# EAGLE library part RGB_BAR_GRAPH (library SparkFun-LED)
SparkFun 48 Segment RGB Bar Graph - Common Anode
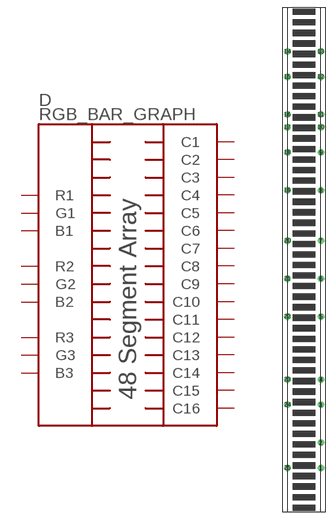
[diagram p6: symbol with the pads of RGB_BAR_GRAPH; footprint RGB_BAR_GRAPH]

Designator prefix D

## RGB_BAR_GRAPHCA (PROD_ID: COM-13520)  [RGB_BAR_GRAPH]
1  C1
2  G3
3  C3
4  C4
5  C6
6  B2
7  G1
8  C10
9  R1
10  C13
11  C14
12  C16
13  R3
14  B3
15  C15
16  G2
17  R2
18  C12
19  C11
20  C9
21  C8
22  C7
23  C5
24  B1
25  C2

## Footprint RGB_BAR_GRAPH (pad centres in mm)
drill 0.8: 1 3.36,-41.9; 2 3.36,-36.82; 3 3.36,-29.2; 4 3.36,-24.12; 5 3.36,-11.42; 6 3.36,-3.8; 7 3.36,3.82; 8 3.36,13.98; 9 3.36,21.6; 10 3.36,26.68; 11 3.36,29.22; 12 3.36,36.84; 13 3.36,41.92; 14 -3.36,41.92; 15 -3.36,36.84; 16 -3.36,29.22; 17 -3.36,26.68; 18 -3.36,21.6; 19 -3.36,13.98; 20 -3.36,3.82; 21 -3.36,-3.8; 22 -3.36,-11.42; 23 -3.36,-24.12; 24 -3.36,-29.2; 25 -3.36,-41.9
